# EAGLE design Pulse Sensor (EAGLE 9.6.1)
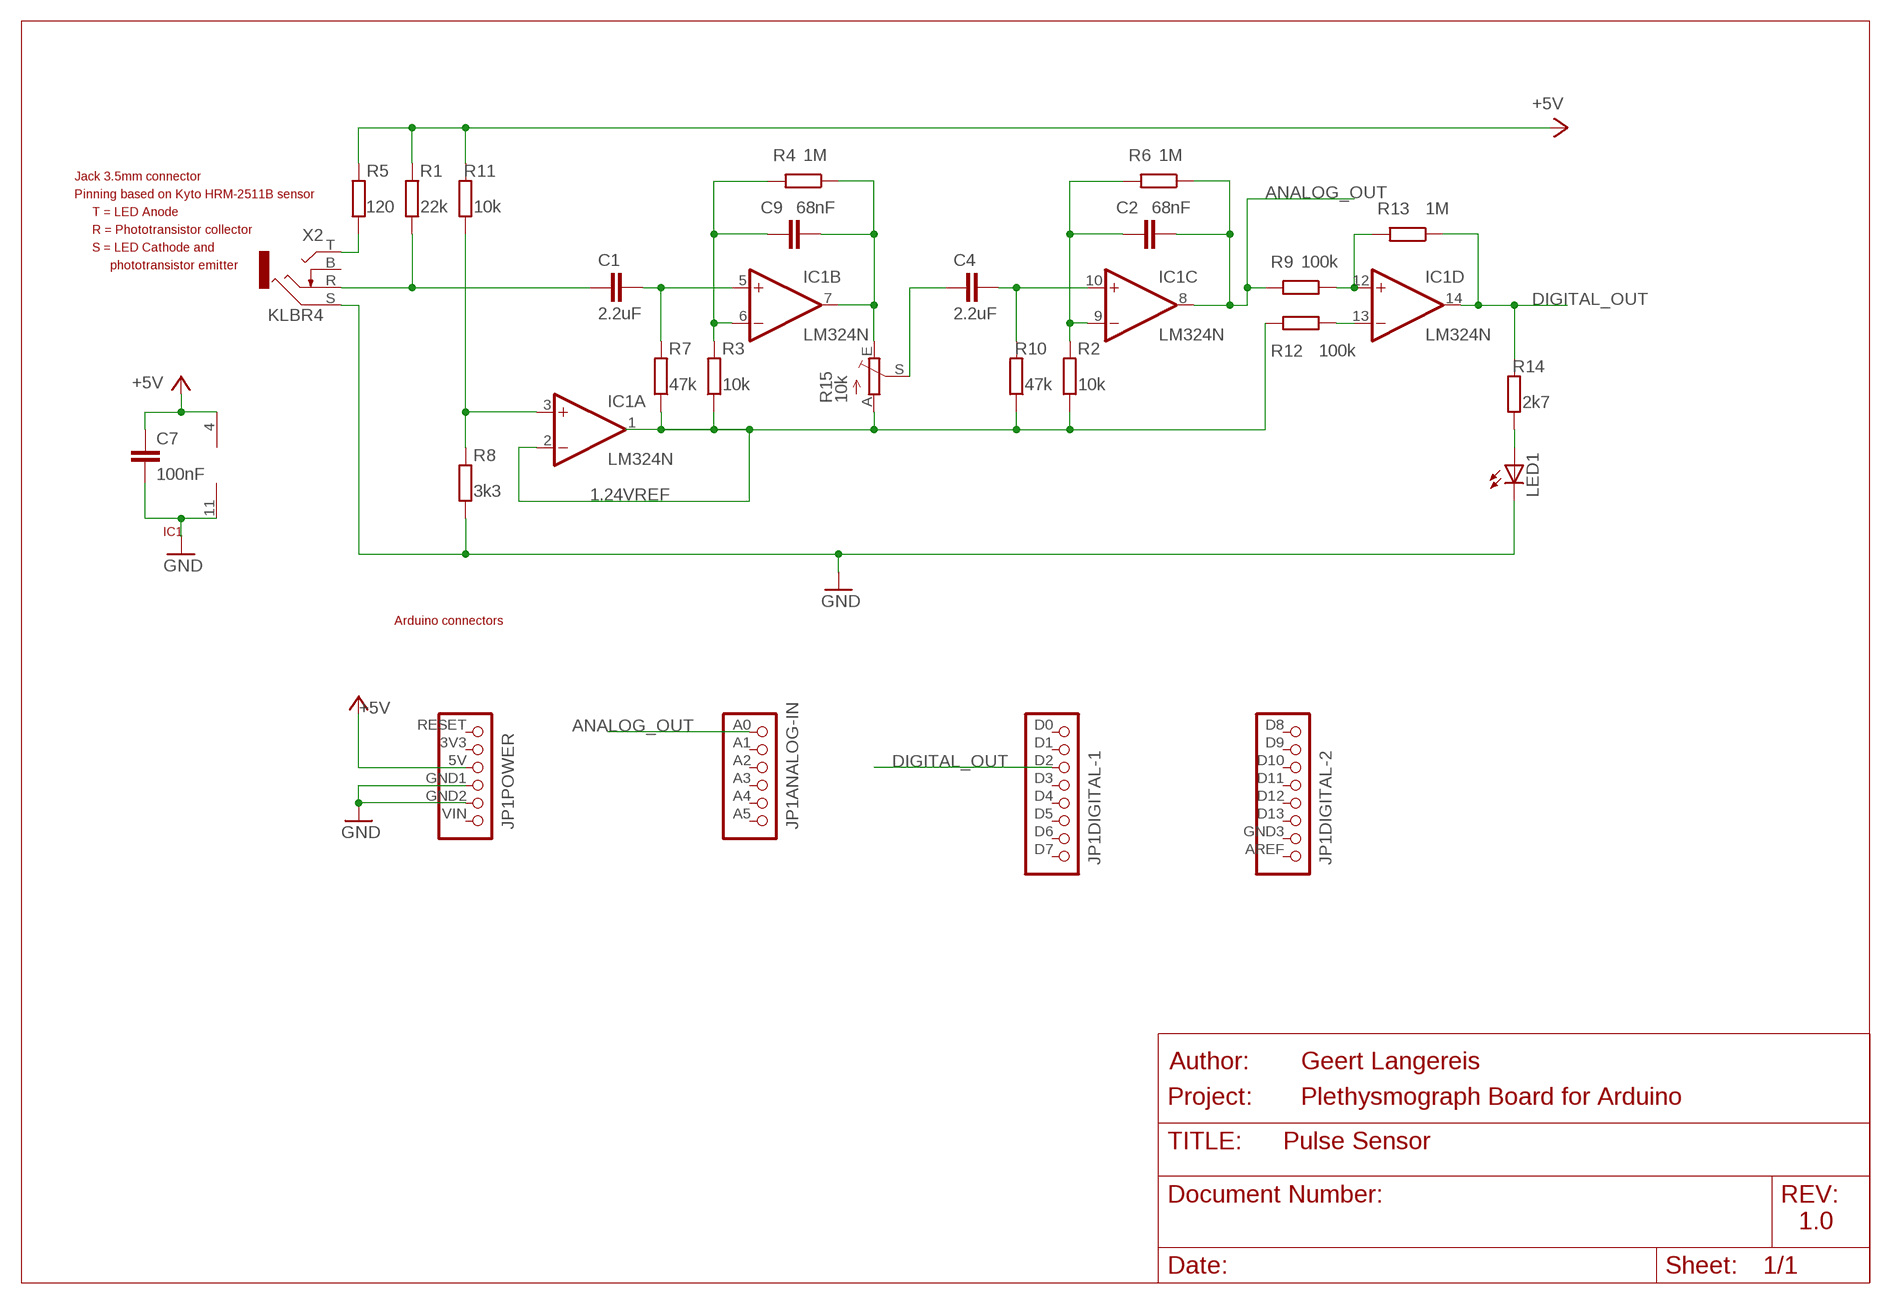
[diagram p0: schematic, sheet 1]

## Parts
C1  2.2uF  C5/7.2  [C5B7.2]
C2  68nF  C5/2.5  [C5B2.5]
C4  2.2uF  C5/7.2  [C5B7.2]
C7  100nF  C5/2.5  [C5B2.5]
C9  68nF  C5/2.5  [C5B2.5]
IC1  LM324N  [DIL14]
JP1  ARDUINO-2009"  [ARDUINO-HEADER]
LED1  LED3MM  [LED3MM]
R1  22k  R-EU_0207/10  [0207/10]
R2  10k  R-EU_0207/10  [0207/10]
R3  10k  R-EU_0207/10  [0207/10]
R4  1M  R-EU_0207/10  [0207/10]
R5  120  R-EU_0207/10  [0207/10]
R6  1M  R-EU_0207/10  [0207/10]
R7  47k  R-EU_0207/10  [0207/10]
R8  3k3  R-EU_0207/10  [0207/10]
R9  100k  R-EU_0207/10  [0207/10]
R10  47k  R-EU_0207/10  [0207/10]
R11  10k  R-EU_0207/10  [0207/10]
R12  100k  R-EU_0207/10  [0207/10]
R13  1M  R-EU_0207/10  [0207/10]
R14  2k7  R-EU_0207/10  [0207/10]
R15  10k  TRIM_EU-S63P  [S63P]
X2  KLBR4  [KLBR4]

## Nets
1.24VREF: IC1.1(A:OUT) IC1.2(A:-IN) R2.1 R3.1 R7.1 R10.1 R12.2 R15.A
+5V: C7.1 IC1.4(P:V+) JP1.5V R1.2 R5.2 R11.2
ANALOG_OUT: C2.2 IC1.8(C:OUT) JP1.A0 R6.1 R9.2
DIGITAL_OUT: IC1.14(D:OUT) JP1.D2 R13.1 R14.2
GND: C7.2 IC1.11(P:V-) JP1.GND1 JP1.GND2 LED1.K(C) R8.1 X2.S
N$1: IC1.12(D:+IN) R9.1 R13.2
N$2: C9.1 IC1.6(B:-IN) R3.2 R4.2
N$3: C9.2 IC1.7(B:OUT) R4.1 R15.E
N$4: IC1.3(A:+IN) R8.2 R11.1
N$5: C4.2 IC1.10(C:+IN) R10.2
N$6: R5.1 X2.T
N$7: C2.1 IC1.9(C:-IN) R2.2 R6.2
N$8: C1.1 R1.1 X2.R
N$9: C1.2 IC1.5(B:+IN) R7.2
N$11: C4.1 R15.S
N$13: IC1.13(D:-IN) R12.1
N$16: LED1.A R14.1
Unconnected: JP1.3V3 JP1.A1 JP1.A2 JP1.A3 JP1.A4 JP1.A5 JP1.AREF JP1.D0 JP1.D1 JP1.D3 JP1.D4 JP1.D5 JP1.D6 JP1.D7 JP1.D8 JP1.D9 JP1.D10 JP1.D11 JP1.D12 JP1.D13 JP1.GND3 JP1.RESET JP1.VIN X2.B

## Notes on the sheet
- Jack 3.5mm connector
- Pinning based on Kyto HRM-2511B sensor
- T = LED Anode
- R = Phototransistor collector
- S = LED Cathode and
- phototransistor emitter
- IC1
- Arduino connectors
- Geert Langereis
- Plethysmograph Board for Arduino
- 1.0

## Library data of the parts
C1 C2 C4 C7 C9 = capacitor-wima:C: CAPACITOR
IC1 = linear:LM324: OP AMP
JP1 = zelf:ARDUINO-2009: Arduino board Arduino Duemilanove
LED1 = led:LED: LED
R1-R14 = rcl:R-EU_: RESISTOR, European symbol
R15 = pot:TRIM_EU-: POTENTIOMETER
X2 = con-lumberg:KLBR4: Jack connectors according to JISC 6560, 3.5 mm Klinkeneinbaukupplung nach JISC 6560, 3,5 mm, 3-polig/ stereo, abgewinkelte Ausführung, mit Öffner, für Leiterplatten Source: Data sheet; MPN: KLBR 4; OC_FARNELL: 1217016; OC_NEWARK: 97K2709

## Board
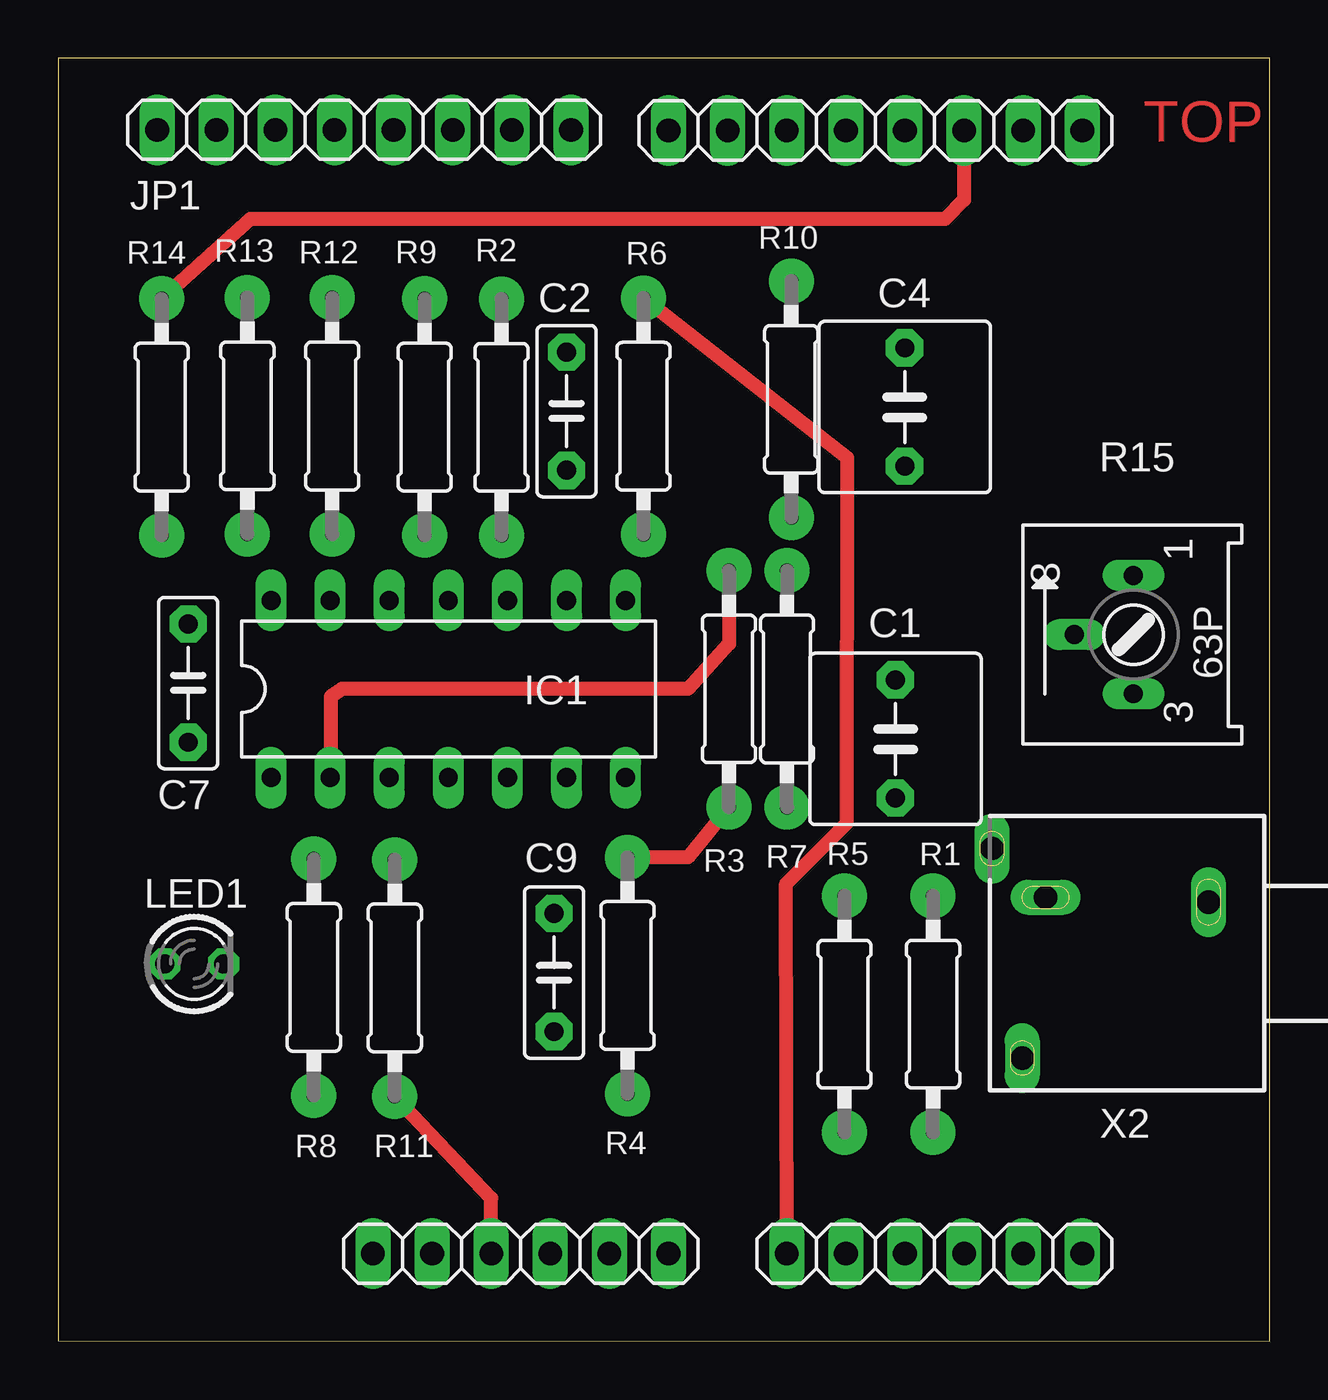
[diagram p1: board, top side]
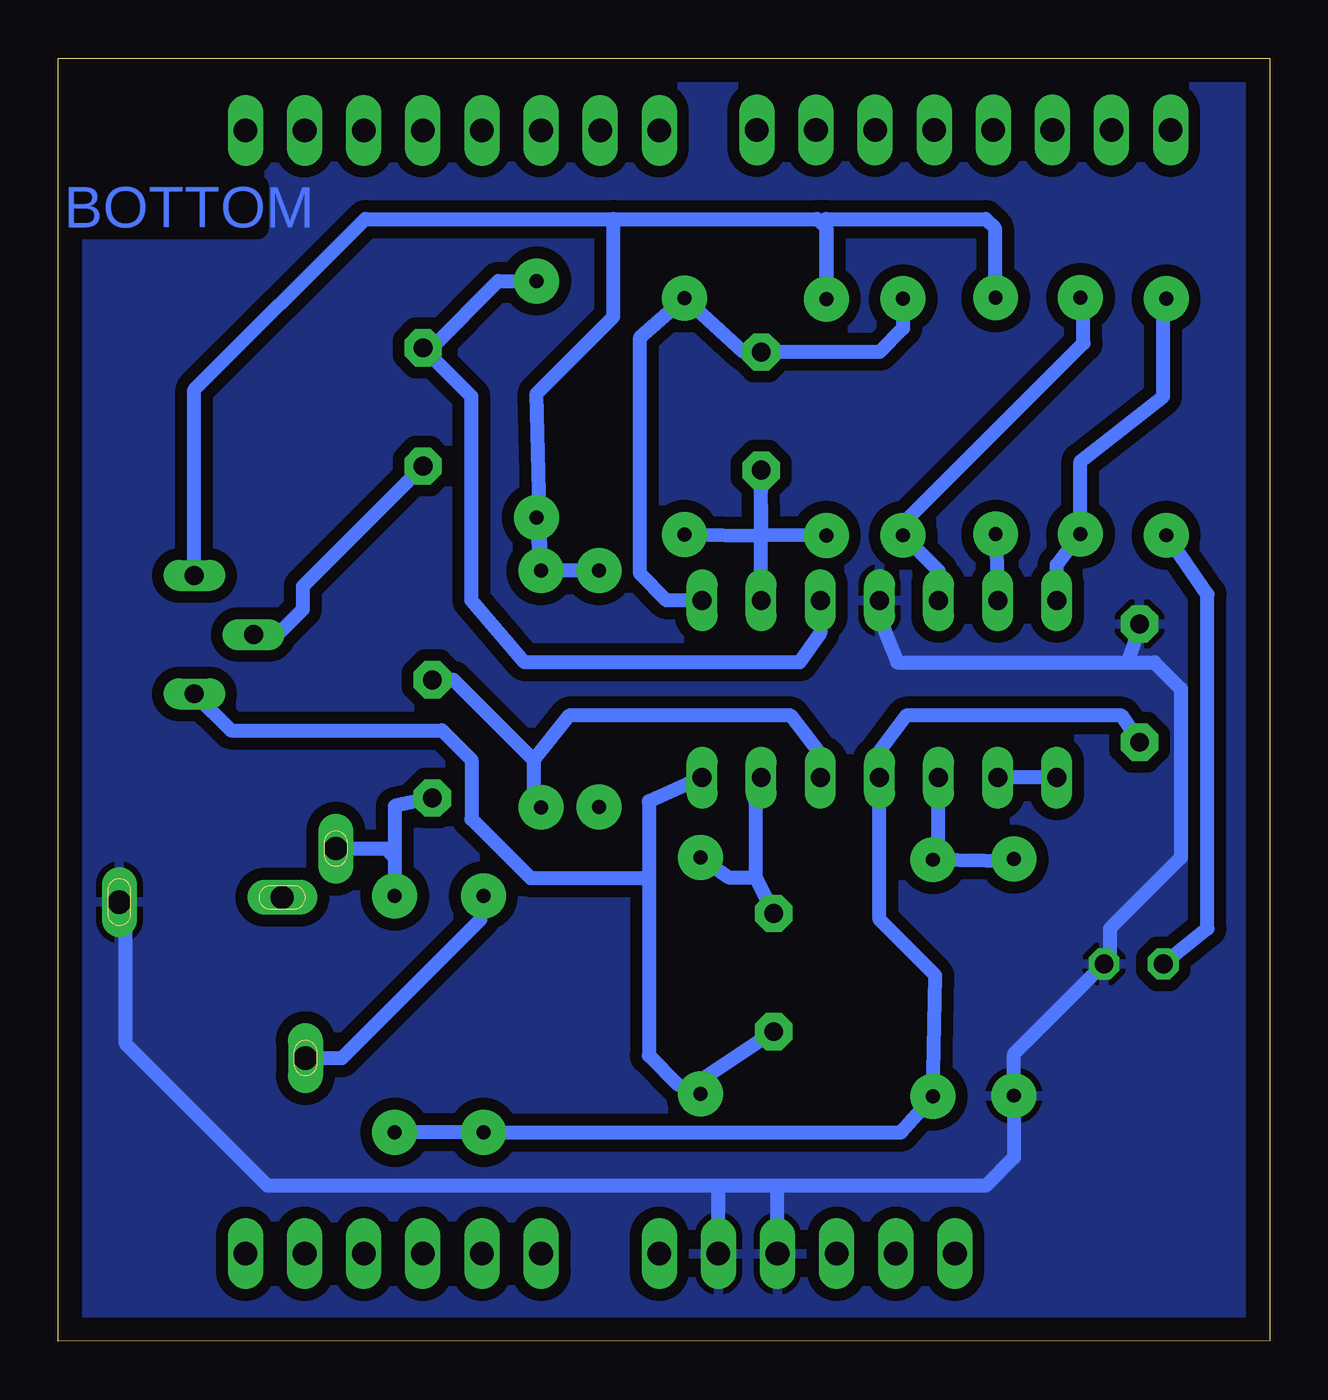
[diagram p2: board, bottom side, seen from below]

Size 52.05 x 55.13 mm. Coordinates in mm from the lower left corner, seen from the top.
Outline: 0,0.02 52.05,0 52.05,55.13 0,55.13 0,0.02
Copper layers (1*16): Top 0.035mm / dielectric 1.5mm / Bottom 0.035mm
Design rules "default *": minimum track width 10mil, minimum drill 24mil, track to track 20mil, track to pad 20mil, pad to pad 20mil, via to via 8mil, smd to smd 8mil, copper to edge 40mil, drill to drill 8mil, minimum pad ring 10mil, minimum via ring 8mil, stop-mask expansion 4mil, vias tented up to drill 0mil, thermal gap 10mil

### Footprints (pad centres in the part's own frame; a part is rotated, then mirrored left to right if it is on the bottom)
C5B7.2 = drill 0.813 pad 1.6 octagon: 1 -2.54,0; 2 2.54,0
C5B2.5 = drill 0.813 pad 1.6 octagon: 1 -2.54,0; 2 2.54,0
DIL14 = drill 0.813 long: 1 -7.62,-3.81; 2 -5.08,-3.81; 3 -2.54,-3.81; 4 0,-3.81; 5 2.54,-3.81; 6 5.08,-3.81; 7 7.62,-3.81; 8 7.62,3.81; 9 5.08,3.81; 10 2.54,3.81; 11 0,3.81; 12 -2.54,3.81; 13 -5.08,3.81; 14 -7.62,3.81
ARDUINO-HEADER = drill 1.016 long: 3V3 2.54,-48.26; 5V 5.08,-48.26; A0 17.78,-48.26; A1 20.32,-48.26; A2 22.86,-48.26; A3 25.4,-48.26; A4 27.94,-48.26; A5 30.48,-48.26; AREF -9.271,0.025; D0 30.48,0; D1 27.94,0; D2 25.4,0; D3 22.86,0; D4 20.32,0; D5 17.78,0; D6 15.24,0; D7 12.7,0; D8 8.509,0.025; D9 5.969,0.025; D10 3.429,0.025; D11 0.889,0.025; D12 -1.651,0.025; D13 -4.191,0.025; GND1 7.62,-48.26; GND2 10.16,-48.26; GND3 -6.731,0.025; RESET 0,-48.26; VIN 12.7,-48.26
LED3MM = drill 0.813 octagon: A -1.27,0; K 1.27,0
0207/10 = drill 0.6 pad 1.93: 1 -5.08,0; 2 5.08,0
S63P = drill 0.813 long: A 2.54,0; E -2.54,0; S 0,2.54
KLBR4 = drill 1 pad 1.3 long: B -2.4,-3.5; S -2.2,3.5 | drill 1 pad 1.2 long: R -4.5,-5.8; T 4.5,-4.5

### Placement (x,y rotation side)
C1  35.98,25.88 90 top
C2  21.84,39.96 90 top
C4  36.37,40.14 90 top
C7  5.59,28.28 90 top
C9  21.31,15.84 270 top
DRILEGEND  [DRILEGEND]  not placed on the board
IC1  16.76,28.03 0 top
JP1  13.52,52.03 0 top
LED1  5.84,16.22 0 top
R1  37.59,14.06 270 top
R2  19.05,39.7 270 top
R3  28.82,28.03 270 top
R4  24.46,15.72 90 top
R5  33.78,14.06 270 top
R6  25.15,39.75 270 top
R7  31.31,28.03 270 top
R8  10.98,15.64 90 top
R9  15.75,39.71 90 top
R10  31.5,40.47 90 top
R11  14.46,15.61 270 top
R12  11.77,39.75 90 top
R13  8.13,39.76 90 top
R14  4.45,39.71 90 top
R15  46.2,30.36 90 top
X2  45.92,16.67 270 top

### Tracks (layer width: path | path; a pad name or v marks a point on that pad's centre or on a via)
1.24VREF
  Top 0.61: R3.1 28.82,29.98 27.05,28.03 12.19,28.03 11.71,27.7 11.71,24.39 IC1.2
  Bottom 0.61: R3.1 R7.1 | IC1.1 IC1.2 | R15.A 46.2,40.88 38.86,48.22 28.19,48.22 | 28.19,48.22 19.43,48.22 19.05,47.84 R2.1 19.05,48.22 12.19,48.22 11.81,47.84 11.81,44.92 R12.2 | R7.1 R10.1 | R7.1 31.5,40.73 28.19,44.03 28.19,48.22
+5V
  Top 0.61: JP1.5V 18.6,6.15 R11.2
  Bottom 0.61: R1.2 R5.2 15.84,8.98 R11.2 14.36,15.72 16.76,18.12 IC1.4 16.76,25.36 15.62,26.88 6.35,26.88 C7.1
ANALOG_OUT
  Top 0.61: JP1.A0 31.27,19.66 33.88,22.27 33.91,37.95 R6.1
  Bottom 0.61: R9.2 15.75,43.52 16.76,42.5 C2.2 22.61,42.5 R6.1 27.05,43.14 27.05,32.98 25.91,31.84 IC1.8
DIGITAL_OUT
  Top 0.61: JP1.D2 38.92,49.04 38.1,48.22 8.26,48.22 R14.2
  Bottom 0.61: IC1.14 9.14,33.36 R13.1 8.13,37.81 4.57,40.6 4.57,44.28 R14.2
GND
  Bottom 0.61: IC1.11 16.76,31.07 16,29.17 6.1,29.17 | 6.1,29.17 5.71,30.31 C7.2 | 21.34,6.69 12.19,6.69 10.98,7.9 R8.1 10.98,12.34 LED1.K 6.86,16.47 6.86,17.74 3.81,20.79 3.81,28.03 4.95,29.17 6.1,29.17 | 21.34,6.69 23.62,6.69 | 23.62,6.69 43.05,6.69 49.15,12.79 49.15,18.6 X2.S | JP1.GND2 23.68,6.63 23.62,6.69 | JP1.GND1 21.14,6.5 21.34,6.69
  pour Bottom: 0.04,54.86 51.75,55.01 51.91,-0.2 -0.04,-0.03
N$1
  Bottom 0.61: R9.1 15.49,34.38 | IC1.12 14.22,33.11 R9.1 | R9.1 15.75,35.14 8,42.89 8,44.41 R13.2
N$2
  Top 0.61: R3.2 27.06,20.8 R4.2
  Bottom 0.61: R4.2 23.24,19.93 22.1,19.93 | 22.1,19.93 C9.1 | IC1.6 22.1,23.2 22.1,19.93
N$3
  Bottom 0.61: C9.2 24.71,11.04 R4.1 25.43,11.04 26.67,12.28 26.67,19.9 | IC1.7 26.67,23.2 26.67,19.9 | R15.E 44.63,26.25 35.56,26.25 34.29,24.98 34.29,22.44 31.75,19.9 26.67,19.9
N$4
  Bottom 0.61: R8.2 11.09,20.62 R11.1 14.22,20.75 IC1.3
N$5
  Bottom 0.61: IC1.10 19.3,30.44 20.19,29.17 32,29.17 34.29,31.84 34.29,40.6 C4.2 36.02,42.68 33.15,45.55 R10.2
N$6
  Bottom 0.61: X2.T 39.86,12.17 33.91,18.12 33.91,19.01 R5.1
N$7
  Bottom 0.61: R6.2 21.78,34.63 21.84,34.88 21.84,34.52 21.85,37.39 | 21.85,37.39 C2.1 | IC1.9 21.86,34.64 | 21.86,34.64 21.84,36.54 21.85,37.39 | R2.2 21.86,34.64
N$8
  Bottom 0.61: C1.1 37.59,22.99 37.59,20.79 | 37.59,20.79 R1.1 | X2.R 37.98,21.17 37.59,20.79
N$9
  Bottom 0.61: IC1.5 19.3,25.23 20.57,26.88 30.1,26.88 31.62,24.98 | 31.62,24.98 31.62,23.07 R7.2 | C1.2 35.07,28.42 31.62,24.98
N$11
  Bottom 0.61: R15.S 42.62,30.36 41.53,31.46 41.53,32.45 C4.1
N$13
  Bottom 0.61: R12.1 IC1.13
N$16
  Bottom 0.61: 4.57,34.63 R14.1 2.67,32.09 2.67,17.74 LED1.A

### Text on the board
Top: TOP
Bottom: BOTTOM
DrillLegend: LAYER-STACK
DrillLegend_01-16: 01-16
